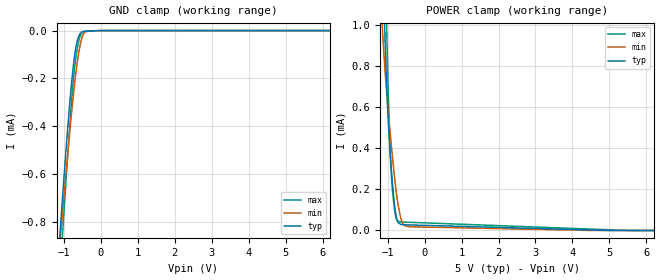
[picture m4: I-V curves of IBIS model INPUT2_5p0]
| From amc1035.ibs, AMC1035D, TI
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|   INPUT2_5p0 Model
[Model]   INPUT2_5p0
Model_type   Input
Vinl = 1.5
Vinh = 3.5
|   typ   min   max
C_comp   2.580E-13   2.509E-13   2.652E-13
|  Where Nom  PVT is Nominal Process,  5.0V,   27C
|   Fast PVT is Strong Process,   5.5V,   -40C
|   Slow PVT is Weak Process,   4.5V,   131C
[Model spec]
|subparameter
Vinl   1.5   1.35   1.65
Vinh   3.5   3.15   3.85
[Voltage Range]   5   4.5   5.5
|Junction Temperature
[Temperature Range]   27   131   -40
[Power Clamp Reference]   5   4.5   5.5
[GND Clamp Reference]   0   0   0
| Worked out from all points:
|   GND clamp passes 1 mA (typ) near -1.17 V on its own axis
|   POWER clamp passes 1 mA (typ) near -1.08 V on its own axis
[GND Clamp]
|   Voltage   I(typ)   I(min)   I(max)
-5V       -10.3mA    -8.279mA   -12.64mA
-1.13V    -902.9uA   -924uA     -1.079mA
-1.085V   -802.5uA   -843.3uA   -968.4uA
-1.04V    -703.8uA   -763.2uA   -858.7uA
-1.025V   -671.3uA   -736.6uA   -822.4uA
-845mV    -309.1uA   -428uA     -404.5uA
-725mV    -122.4uA   -242.4uA   -175.7uA
-680mV    -74.73uA   -182uA     -117.6uA
-605mV    -26.71uA   -98.64uA   -48.61uA
-485mV    -4.033uA   -18.2uA    -6.017uA
-5mV      -16.78nA   -9.854nA   -25.85nA
10V       0A         0A         0A
[POWER Clamp]
|   Voltage   I(typ)   I(min)   I(max)
-5V       36.45mA    27.6mA     45.68mA
-1.16V    1.515mA    1.047mA    2.226mA
-1.13V    1.305mA    945.9uA    1.93mA
-1.085V   1.016mA    815.5uA    1.502mA
-1.025V   699.7uA    669.6uA    978.6uA
-950mV    426.7uA    511uA      471.6uA
-890mV    272uA      394.5uA    242.7uA
-800mV    103.1uA    237.2uA    84.53uA
-740mV    46.97uA    150.8uA    48.6uA
-650mV    29.4uA     63.2uA     41.82uA
-410mV    27.04uA    18.22uA    39.92uA
10V       0A         0A         0A
